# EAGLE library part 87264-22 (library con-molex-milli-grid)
RECEPTACAL
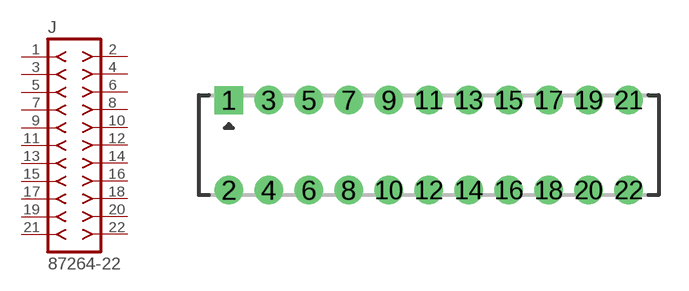
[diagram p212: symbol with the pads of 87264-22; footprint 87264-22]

Designator prefix J

## 87264-22  [87264-22]
1  1  pas
2  2  pas
3  3  pas
4  4  pas
5  5  pas
6  6  pas
7  7  pas
8  8  pas
9  9  pas
10  10  pas
11  11  pas
12  12  pas
13  13  pas
14  14  pas
15  15  pas
16  16  pas
17  17  pas
18  18  pas
19  19  pas
20  20  pas
21  21  pas
22  22  pas

## Footprint 87264-22 (pad centres in mm)
RECEPTACAL Dual Row, Side Entry
drill 0.914 square: 1 -10,2.25
drill 0.914: 2 -10,-2.25; 3 -8,2.25; 4 -8,-2.25; 5 -6,2.25; 6 -6,-2.25; 7 -4,2.25; 8 -4,-2.25; 9 -2,2.25; 10 -2,-2.25; 11 0,2.25; 12 0,-2.25; 13 2,2.25; 14 2,-2.25; 15 4,2.25; 16 4,-2.25; 17 6,2.25; 18 6,-2.25; 19 8,2.25; 20 8,-2.25; 21 10,2.25; 22 10,-2.25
